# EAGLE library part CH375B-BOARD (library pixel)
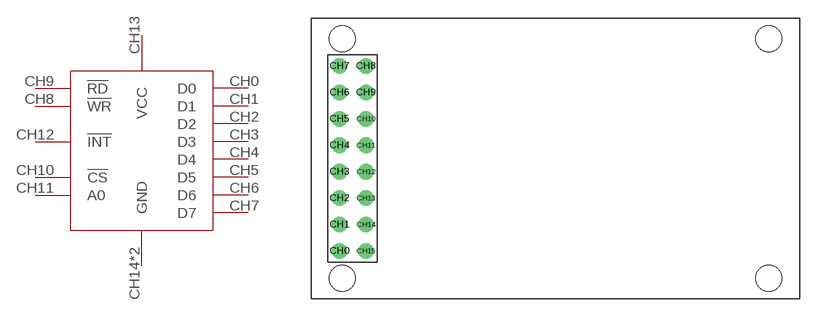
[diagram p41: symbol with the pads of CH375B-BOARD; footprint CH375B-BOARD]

Designator prefix -

## CH375B-BOARD  [CH375B-BOARD]
CH0  D0
CH1  D1
CH2  D2
CH3  D3
CH4  D4
CH5  D5
CH6  D6
CH7  D7
CH8  !WR
CH9  !RD
CH10  !CS
CH11  A0
CH12  !INT
CH13  VCC
CH14  GND
CH15  GND

## Footprint CH375B-BOARD (pad centres in mm)
drill 1: CH0 -1.27,-8.89; CH1 -1.27,-6.35; CH2 -1.27,-3.81; CH3 -1.27,-1.27; CH4 -1.27,1.27; CH5 -1.27,3.81; CH6 -1.27,6.35; CH7 -1.27,8.89; CH8 1.27,8.89; CH9 1.27,6.35; CH10 1.27,3.81; CH11 1.27,1.27; CH12 1.27,-1.27; CH13 1.27,-3.81; CH14 1.27,-6.35; CH15 1.27,-8.89
hole 2.5 at -1,11.5
hole 2.5 at -1,-11.5
hole 2.5 at 40,11.5
hole 2.5 at 40,-11.5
